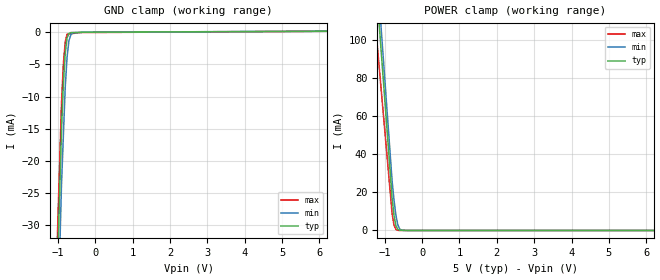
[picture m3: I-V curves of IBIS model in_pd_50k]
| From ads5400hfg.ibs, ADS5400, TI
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[Model] in_pd_50k
Model_type Input
Vinl = 800.000mV
Vinh = 2.00000V
C_comp 520.000fF 513.000fF 554.000fF
| variable typ   min   max
[Voltage Range] 5.00000V 4.75000V 5.25000V
[POWER Clamp Reference] 5.00000V 4.75000V 5.25000V
[GND Clamp Reference] 0.00000V 0.00000V 0.00000V
[Temperature Range] 25   85   -40
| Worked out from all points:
|   GND clamp passes 1 mA (typ) near -0.75 V on its own axis
|   POWER clamp passes 1 mA (typ) near -0.66 V on its own axis
[GND Clamp]
-5V       -838.9mA   -916.8mA   -780.6mA
-900mV    -15.25mA   -23.7mA    -11.08mA
-850mV    -8.101mA   -16.13mA   -4.968mA
-800mV    -3.304mA   -8.556mA   -1.513mA
-750mV    -909uA     -3.854mA   -305.2uA
-700mV    -197.3uA   -1.312mA   -272.3uA
-650mV    -58.06uA   -396.6uA   -239.4uA
-600mV    -50.64uA   -102uA     -206.5uA
-375mV    -17.27uA   -32.4uA    -58.45uA
-325mV    -9.849uA   -16.94uA   -56.93uA
-300mV    -9.257uA   -9.213uA   -56.18uA
10V       234.9uA    242.3uA    255.6uA
[POWER Clamp]
-5V       1.122A     1.173A     941.5mA
-1.05V    82.78mA    94.19mA    64.43mA
-800mV    17.01mA    25.88mA    8.916mA
-750mV    7.935mA    16.12mA    2.876mA
-700mV    2.681mA    8.082mA    580.2uA
-650mV    606uA      3.091mA    114.2uA
-600mV    106.6uA    879.6uA    21.83uA
-500mV    71.08uA    34.49uA    16.69uA
10V       0A         0A         0A
